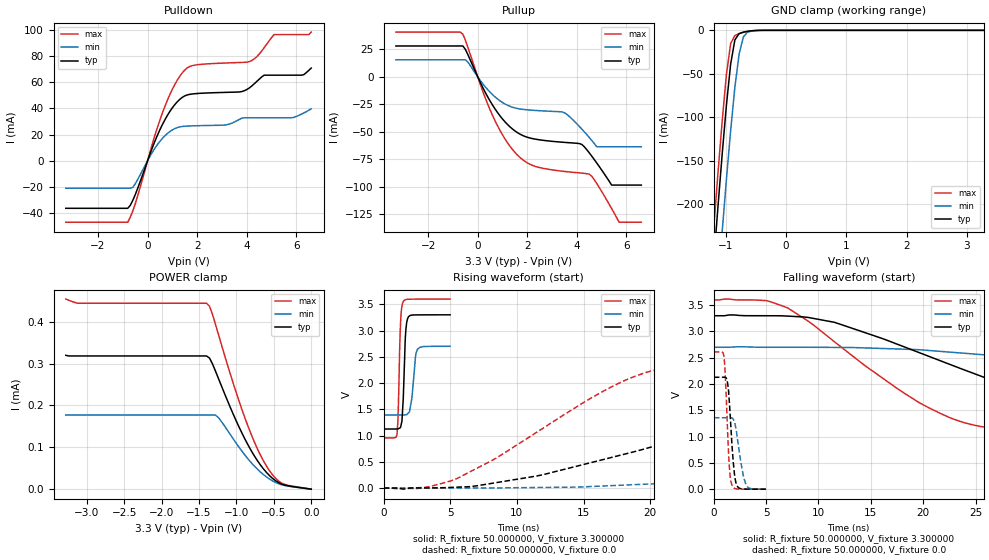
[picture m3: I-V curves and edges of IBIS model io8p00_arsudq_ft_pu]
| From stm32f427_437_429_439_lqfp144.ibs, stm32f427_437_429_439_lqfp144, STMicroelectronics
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|   Model io8p00_arsudq_ft_pu
[Model]  io8p00_arsudq_ft_pu
Model_type I/O
Polarity   Non-Inverting
Enable   Active-Low
Vinl =   0.990000V
Vinh =   2.310000V
Vmeas =  1.650000V
Cref =   50.000000pF
Rref =   100.000000M
Vref =   0.0V
C_comp   2.292100pF   2.228000pF   2.366600pF
[Temperature Range]   25.000000   0.125000k   -40.000000
[Pullup Reference]   3.300000V   2.700000V   3.600000V
[Pulldown Reference]   0.0V   0.0V   0.0V
[POWER Clamp Reference]   3.300000V   2.700000V   3.600000V
[GND Clamp Reference]   0.0V   0.0V   0.0V
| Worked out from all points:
|   slope of the pulldown table from 0 to 0.495 V, typ, clamps not added: 20.9 ohm
|   slope of the pullup table from 0 to 0.495 V, typ, clamps not added: 22.6 ohm
|   GND clamp passes 1 mA (typ) near -0.62 V on its own axis
|   rising waveform, R_fixture 50.000000, V_fixture 3.300000: 20-80 % time 190ps typ, 291ps min, 164ps max; typ from 1.12 V to 3.3 V
|   rising waveform, R_fixture 50.000000, V_fixture 0.0: 20-80 % time 19.7ns typ, 51ns min, 10.4ns max; typ from 0.001 V to 2.13 V
|   falling waveform, R_fixture 50.000000, V_fixture 3.300000: 20-80 % time 18.9ns typ, 44.4ns min, 11.4ns max; typ from 3.3 V to 1.12 V
|   falling waveform, R_fixture 50.000000, V_fixture 0.0: 20-80 % time 433ps typ, 633ps min, 343ps max; typ from 2.13 V to 0.001 V
[Pulldown]
|Voltage   I(typ)   I(min)   I(max)
-3.3V     -36.46mA   -21.09mA   -47.09mA
-800mV    -36.46mA   -21.09mA   -47.09mA
-600mV    -30.5mA    -20.55mA   -38.69mA
700mV     31.4mA     19.11mA    41.71mA
1.2V      45.15mA    25.37mA    61.75mA
1.6V      50.35mA    26.5mA     71.06mA
3.1V      52.28mA    27.26mA    74.76mA
4.1V      55.64mA    32.87mA    75.8mA
4.7V      65.47mA    32.87mA    86.49mA
5.1V      65.47mA    32.87mA    96.56mA
6.2V      65.47mA    35.57mA    96.56mA
6.6V      70.92mA    39.71mA    98.46mA
[Pullup]
|Voltage   I(typ)   I(min)   I(max)
-3.3V     28.01mA    15.42mA    40.63mA
-700mV    28.01mA    15.42mA    40.63mA
-400mV    20.31mA    13.47mA    26.93mA
600mV     -25.77mA   -16.23mA   -35.13mA
1.6V      -50.64mA   -28.8mA    -70.96mA
3.5V      -59.52mA   -32.65mA   -85.91mA
4.2V      -61.43mA   -47.48mA   -87.45mA
4.5V      -69.07mA   -55.12mA   -88.37mA
4.8V      -78.22mA   -63.5mA    -96.83mA
5.4V      -98.3mA    -63.5mA    -119.6mA
5.7V      -98.3mA    -63.5mA    -132mA
6.6V      -98.3mA    -63.5mA    -132mA
[GND_clamp]
|Voltage   I(typ)   I(min)   I(max)
-3.3V     -2.319A    -2.398A    -2.292A
-1.2V     -265.5mA   -356.1mA   -227.2mA
-1.13V    -202.6mA   -292.9mA   -164.1mA
-1.06V    -142.2mA   -231.2mA   -104.1mA
-990mV    -85.98mA   -171.6mA   -50.72mA
-920mV    -38.8mA    -115.5mA   -15.28mA
-850mV    -11.08mA   -65.6mA    -6.001mA
-780mV    -3.782mA   -27.42mA   -3.876mA
-710mV    -2.086mA   -7.69mA    -2.381mA
-640mV    -1.147mA   -2.118mA   -1.22mA
-570mV    -523.9uA   -798.4uA   -476.8uA
3.28V     0A         0A         0A
[POWER_clamp]
|Voltage   I(typ)   I(min)   I(max)
-3.28V    319.9uA    177.1uA    454.3uA
-3.12V    318.3uA    177.1uA    444.3uA
-1.4V     318.3uA    177.1uA    444.3uA
-1.36V    313.4uA    177.1uA    437.2uA
-1.28V    282.3uA    177.1uA    394.1uA
-1.24V    264.6uA    170.9uA    369.7uA
-920mV    131.9uA    89.35uA    187.2uA
-760mV    79.47uA    55.13uA    112.7uA
-640mV    48.78uA    35.04uA    68.06uA
-520mV    26.21uA    20.11uA    35uA
-400mV    12.52uA    10.81uA    14.88uA
0V        0A         0A         0A
[Ramp]
| variable   typ   min   max
dV/dt_r  1.27717/19.70736n   0.81531/51.01041n   1.56688/10.34395n
dV/dt_f  1.30524/18.83539n   0.78426/44.46831n   1.58714/11.33778n
R_load = 50.000000
[Rising Waveform]
R_fixture= 50.000000
V_fixture= 3.300000
V_fixture_min= 2.700000
V_fixture_max= 3.600000
|time   V(typ)   V(min)   V(max)
0s        1.125V     1.393V     954.7mV
1.001ns   1.127V     1.393V     1.019V
1.071ns   1.129V     1.393V     1.29V
1.281ns   1.171V     1.393V     3.209V
1.461ns   1.663V     1.392V     3.546V
1.632ns   2.886V     1.395V     3.589V
1.862ns   3.261V     1.432V     3.596V
2.112ns   3.294V     1.704V     3.598V
2.533ns   3.298V     2.642V     3.599V
4.985ns   3.3V       2.7V       3.6V
[Rising Waveform]
R_fixture= 50.000000
V_fixture= 0.0
V_fixture_min= 0.0
V_fixture_max= 0.0
|time   V(typ)   V(min)   V(max)
0s        1.088mV    1.043mV    1.136mV
5.506ns   17.83mV    2.783mV    182.4mV
11.51ns   231.1mV    11.16mV    1.067V
19.02ns   706.8mV    67.68mV    2.143V
27.53ns   1.301V     166.1mV    2.489V
38.04ns   1.843V     353.7mV    2.576V
57.06ns   2.067V     702.7mV    2.609V
89.09ns   2.119V     1.141V     2.613V
117.6ns   2.129V     1.3V       2.613V
249.2ns   2.13V      1.36V      2.613V
[Falling Waveform]
R_fixture= 50.000000
V_fixture= 3.300000
V_fixture_min= 2.700000
V_fixture_max= 3.600000
|time   V(typ)   V(min)   V(max)
0s        3.3V       2.7V       3.6V
5.506ns   3.3V       2.7V       3.561V
11.51ns   3.175V     2.697V     2.806V
22.52ns   2.376V     2.608V     1.363V
31.53ns   1.726V     2.431V     1.075V
41.04ns   1.36V      2.21V      1.014V
49.55ns   1.249V     2.021V     991.5mV
81.58ns   1.151V     1.586V     958.3mV
106.6ns   1.134V     1.464V     955.9mV
249.2ns   1.125V     1.393V     954.7mV
[Falling Waveform]
R_fixture= 50.000000
V_fixture= 0.0
V_fixture_min= 0.0
V_fixture_max= 0.0
|time   V(typ)   V(min)   V(max)
0s        2.13V      1.36V      2.613V
981ps     2.131V     1.36V      2.507V
1.151ns   2.121V     1.359V     1.945V
1.411ns   1.87V      1.36V      683.4mV
1.542ns   1.488V     1.362V     294.8mV
1.742ns   830.4mV    1.355V     76.08mV
2.152ns   99.77mV    1.12V      7.624mV
2.573ns   10.56mV    525.8mV    2.036mV
3.123ns   1.941mV    73.6mV     1.207mV
4.985ns   1.088mV    1.043mV    1.136mV
